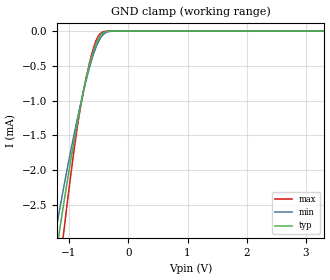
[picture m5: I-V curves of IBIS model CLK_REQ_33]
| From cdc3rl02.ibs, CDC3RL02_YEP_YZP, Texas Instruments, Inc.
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[Model]   CLK_REQ_33
Model_type  Input
Vinl=0.5
Vinh=1.3
| variable   typ   min   max
C_comp   1.89pF   1.30pF   2.08pF
[Temperature Range]   40   100   -40
| Ambient temperature   25   85   -40
[Voltage range]   3.3   3   3.6
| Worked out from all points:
|   GND clamp passes 1 mA (typ) near -0.79 V on its own axis
[GND Clamp]
| CLK_REQ_33
|   Voltage   I(typ)   I(min)   I(max)
-3.3V     -17.89mA   -15.4mA    -22.19mA
-1.245V   -3.357mA   -2.981mA   -4.04mA
-1.21V    -3.155mA   -2.811mA   -3.776mA
-1.175V   -2.955mA   -2.643mA   -3.514mA
-1.11V    -2.593mA   -2.339mA   -3.038mA
-1.08V    -2.429mA   -2.201mA   -2.823mA
-875mV    -1.387mA   -1.321mA   -1.468mA
-730mV    -754.9uA   -774.3uA   -751.9uA
-575mV    -259.5uA   -302.8uA   -210.2uA
-435mV    -32.9uA    -61.02uA   -14.38uA
-245mV    -197.4nA   -1.106uA   -12.45nA
3.3V      134pA      16.57nA    74.46pA
